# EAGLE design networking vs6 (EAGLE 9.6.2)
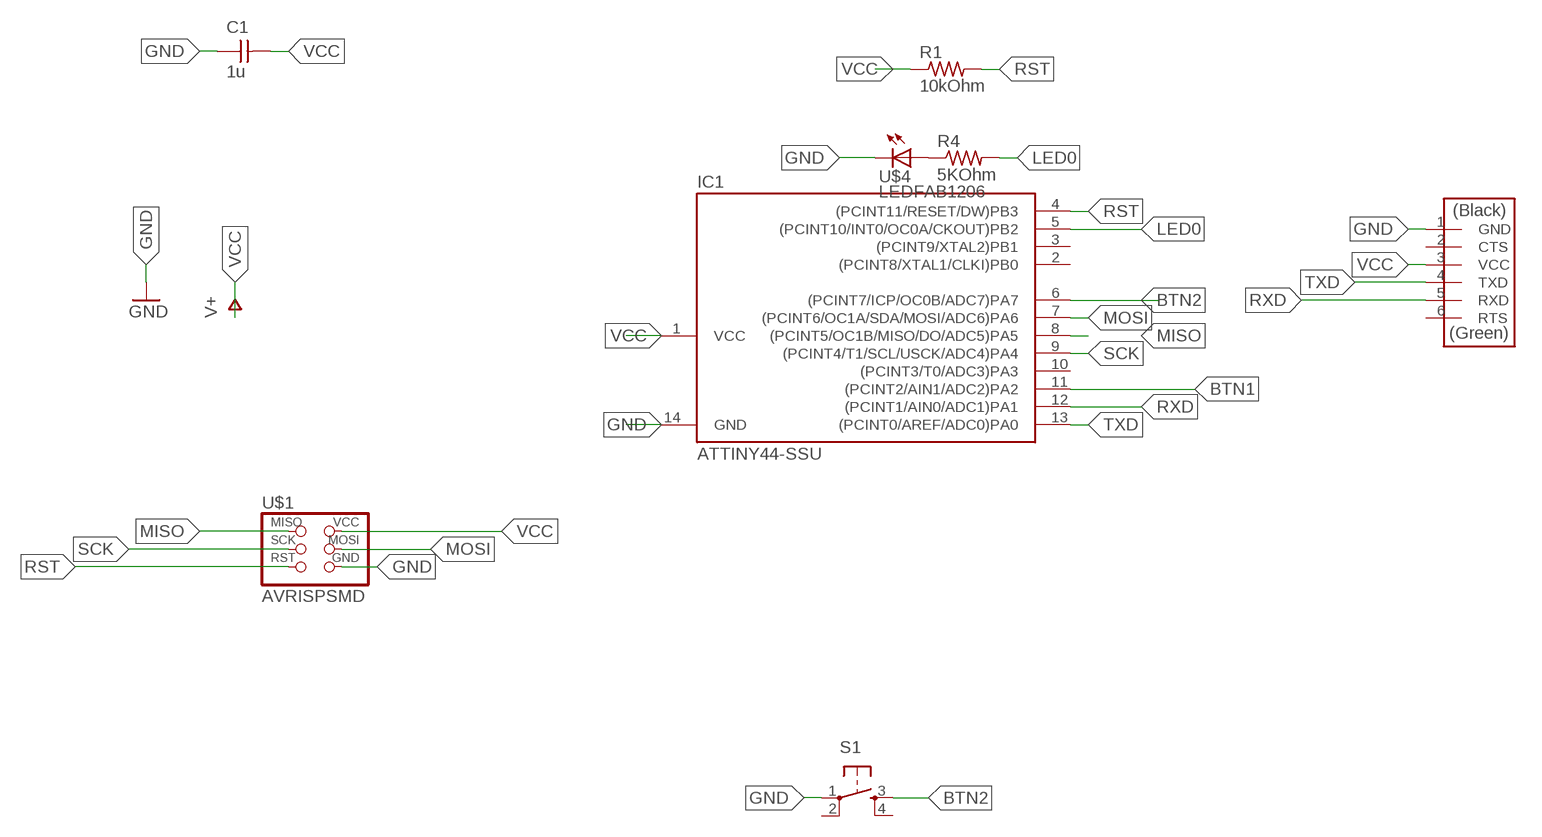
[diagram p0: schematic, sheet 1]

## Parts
C1  1u  CAP-UNPOLARIZEDFAB  [C1206FAB]
IC1  ATTINY44-SSU  [SOIC14]
R1  10kOhm  RES-US1206FAB  [R1206FAB]
R4  5KOhm  RES-US1206FAB  [R1206FAB]
S1  6MM_SWITCH6MM_SWITCH  [6MM_SWITCH]
U$1  AVRISPSMD  [2X03SMD]
U$2  FTDI-SMD-HEADER  [1X06SMD]
U$4  LEDFAB1206  [LED1206FAB]

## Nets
BTN1: IC1.11((PCINT2/AIN1/ADC2)PA2)
BTN2: IC1.6((PCINT7/ICP/OC0B/ADC7)PA7) S1.3(S)
GND: C1.1 IC1.14(GND) S1.1(P) U$1.6(GND) U$2.1(GND) U$4.2(C)
LED0: IC1.5((PCINT10/INT0/OC0A/CKOUT)PB2) R4.2
MISO: IC1.8((PCINT5/OC1B/MISO/DO/ADC5)PA5) U$1.1(MISO)
MOSI: IC1.7((PCINT6/OC1A/SDA/MOSI/ADC6)PA6) U$1.4(MOSI)
N$1: R4.1 U$4.1(A)
RST: IC1.4((PCINT11/RESET/DW)PB3) R1.2 U$1.5(RST)
RXD: IC1.12((PCINT1/AIN0/ADC1)PA1) U$2.5(RXD)
SCK: IC1.9((PCINT4/T1/SCL/USCK/ADC4)PA4) U$1.3(SCK)
TXD: IC1.13((PCINT0/AREF/ADC0)PA0) U$2.4(TXD)
VCC: C1.2 IC1.1(VCC) R1.1 U$1.2(VCC) U$2.3(VCC) ; supply symbol labelled V+
Unconnected: IC1.2((PCINT8/XTAL1/CLKI)PB0) IC1.3((PCINT9/XTAL2)PB1) IC1.10((PCINT3/T0/ADC3)PA3) S1.2(P1) S1.4(S1) U$2.2(CTS) U$2.6(RTS)

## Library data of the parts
C1 = fab:CAP-UNPOLARIZED
IC1 = fab:ATTINY44
R1 R4 = fab:RES-US: Resistor (US Symbol)
S1 = fab:6MM_SWITCH: OMRON SWITCH
U$1 = fab:AVRISP
U$2 = fab:FTDI-SMD-HEADER
U$4 = fab:LED: LED

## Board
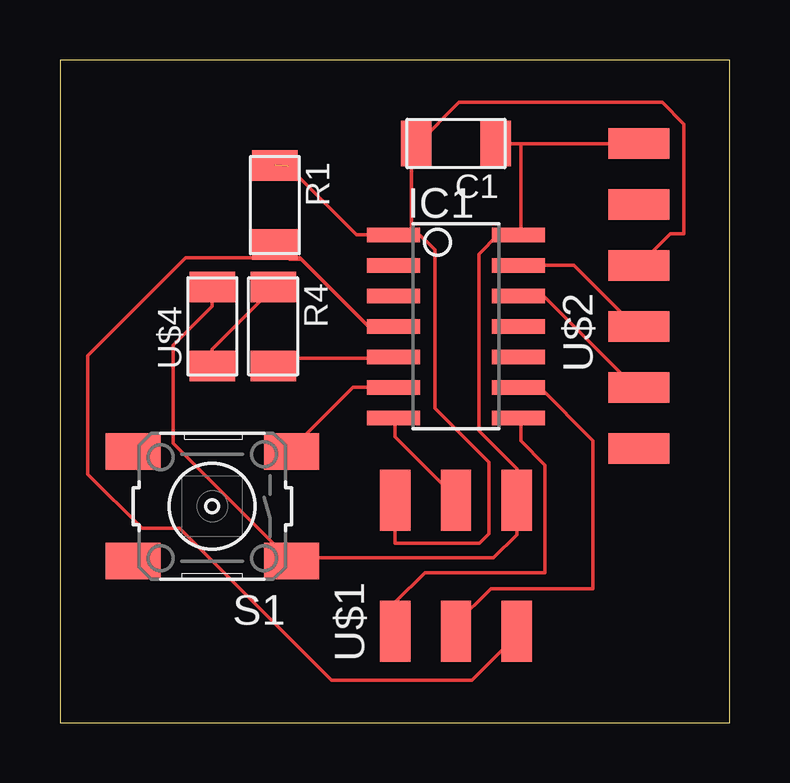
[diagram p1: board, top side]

Size 27.92 x 27.61 mm. Coordinates in mm from the lower left corner, seen from the top.
Outline: 0,0 27.92,0 27.92,27.61 0,27.61 0,0
Copper layers (1*16): Top 0.035mm / dielectric 1.5mm / Bottom 0.035mm
Design rules "default *": minimum track width 6mil, minimum drill 0.35mm, track to track 17mil, track to pad 17mil, pad to pad 6mil, via to via 6mil, smd to smd 6mil, copper to edge 40mil, drill to drill 6mil, minimum pad ring 10mil, minimum via ring 8mil, stop-mask expansion 4mil, vias tented up to drill 0mil, thermal gap 10mil

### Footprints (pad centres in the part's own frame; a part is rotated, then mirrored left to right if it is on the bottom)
C1206FAB = smd 1.27 x 1.905: 1 -1.651,0; 2 1.651,0
SOIC14 = smd 0.61 x 2.21: 1 -3.81,-2.603; 2 -2.54,-2.603; 3 -1.27,-2.603; 4 0,-2.603; 5 1.27,-2.603; 6 2.54,-2.603; 7 3.81,-2.603; 8 3.81,2.603; 9 2.54,2.603; 10 1.27,2.603; 11 0,2.603; 12 -1.27,2.603; 13 -2.54,2.603; 14 -3.81,2.603
R1206FAB = smd 1.27 x 1.905: 1 -1.651,0; 2 1.651,0
6MM_SWITCH = smd 2.286 x 1.524: 1 -3.302,2.286; 2 3.302,2.286; 3 -3.302,-2.286; 4 3.302,-2.286
2X03SMD = smd 2.54 x 1.27: 1 -2.54,2.54; 2 2.92,2.54; 3 -2.54,0; 4 2.92,0; 5 -2.54,-2.54; 6 2.92,-2.54
1X06SMD = smd 2.54 x 1.27: 1 0,6.35; 2 0,3.81; 3 0,1.27; 4 0,-1.27; 5 0,-3.81; 6 0,-6.35
LED1206FAB = smd 1.27 x 1.905: 1 -1.651,0; 2 1.651,0

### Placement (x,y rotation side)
C1  16.51,24.13 180 top
IC1  16.51,16.51 270 top
R1  8.96,21.57 270 top
R4  8.89,16.51 270 top
S1  6.35,9.02 180 top
U$1  16.51,6.35 90 top
U$2  24.13,17.78 0 top
U$4  6.35,16.51 90 top

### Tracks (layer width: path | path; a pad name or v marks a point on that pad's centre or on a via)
BTN2
  Top 0.152: IC1.6 12.22,13.97 9.68,11.43 S1.3
GND
  Top 0.152: U$2.1 19.21,24.13 | 19.21,24.13 C1.1 | 19.21,24.13 19.21,20.32 IC1.14 18.26,20.32 17.46,19.53 17.46,12.17 19.05,10.58 U$1.6 19.05,7.83 18.08,6.86 9.78,6.86 S1.1 9.53,6.83 4.72,11.63 4.72,15.72 6.35,17.35 U$4.2
LED0
  Top 0.152: R4.2 8.89,15.18 13.75,15.18 13.81,15.24 IC1.5
MISO
  Top 0.152: U$1.1 13.97,5.01 15.22,6.25 20.23,6.25 20.23,10.73 19.21,11.75 19.21,12.7 IC1.8
MOSI
  Top 0.152: IC1.7 13.97,12.7 13.97,11.91 16.51,9.37 U$1.4
N$1
  Top 0.152: U$4.1 6.35,15.56 8.89,18.1 R4.1
RST
  Top 0.152: 12.86,16.51 IC1.4 | 12.86,16.51 10,19.37 5.24,19.37 1.16,15.29 1.16,10.36 3.43,8.1 4.99,8.1 11.32,1.77 17.17,1.77 19.05,3.65 U$1.5 | R1.2 9.57,19.3 10.05,19.3 12.85,16.51 12.86,16.51
RXD
  Top 0.152: IC1.12 20.16,17.78 23.97,13.97 U$2.5
SCK
  Top 0.152: IC1.9 20,13.97 22.22,11.75 22.22,5.59 17.97,5.59 16.51,4.13 U$1.3
TXD
  Top 0.152: IC1.13 21.43,19.05 23.97,16.51 U$2.4
VCC  (1 unrouted)
  Top 0.152: 14.66,20.3 14.66,24.13 C1.2 14.92,24.13 16.64,25.84 25.11,25.84 26.02,24.94 26.02,20.38 25.46,20.38 U$2.3 | 14.66,20.3 14.68,20.27 14.86,20.46 15.62,19.7 15.62,13.11 17.88,10.86 17.88,7.87 17.48,7.47 13.97,7.47 U$1.2 | 14.66,20.3 14.65,20.31 14.64,20.32 IC1.1 12.37,20.32 9.52,23.17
